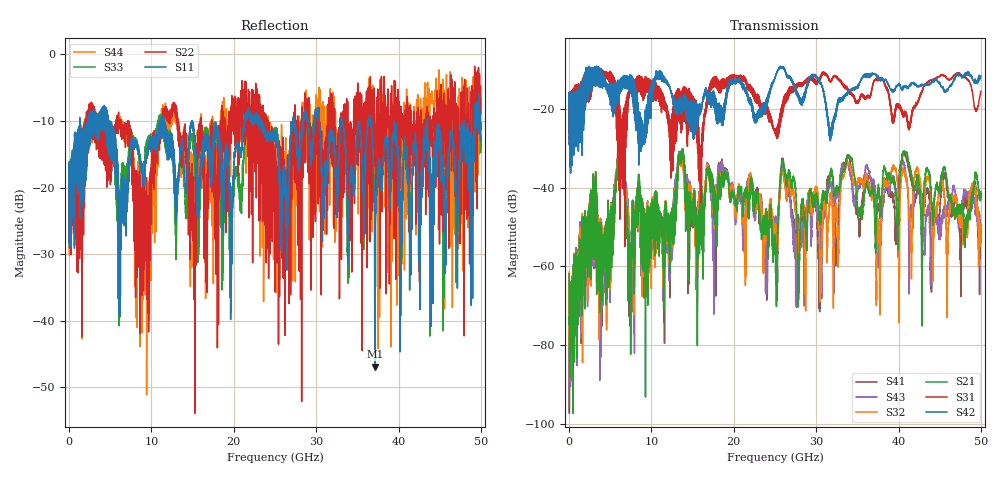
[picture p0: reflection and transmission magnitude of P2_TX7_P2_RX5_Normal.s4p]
!Keysight Technologies,N5225B,MY57041031,A.13.20.10
!Date: Friday, May 31, 2019 11:34:46
!Correction: S11(Full 4 Port(1,2,3,4))
!S12(Full 4 Port(1,2,3,4))
!S13(Full 4 Port(1,2,3,4))
!S14(Full 4 Port(1,2,3,4))
!S21(Full 4 Port(1,2,3,4))
!S22(Full 4 Port(1,2,3,4))
!S23(Full 4 Port(1,2,3,4))
!S24(Full 4 Port(1,2,3,4))
!S31(Full 4 Port(1,2,3,4))
!S32(Full 4 Port(1,2,3,4))
!S33(Full 4 Port(1,2,3,4))
!S34(Full 4 Port(1,2,3,4))
!S41(Full 4 Port(1,2,3,4))
!S42(Full 4 Port(1,2,3,4))
!S43(Full 4 Port(1,2,3,4))
!S44(Full 4 Port(1,2,3,4))
!S4P File: Measurements: <S11,S12,S13,S14>,
!<S21,S22,S23,S24>,
!<S31,S32,S33,S34>,
!<S41,S42,S43,S44>:
# Hz S  dB  R 50.0
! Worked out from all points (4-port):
!   5000 points, 10 MHz to 50 GHz, reference 50 ohm
!   strongest paths, dB at 10 MHz, 12.51 GHz, 25.01 GHz, 37.51 GHz, 50 GHz:
!     S42: -19.4, -16.9, -11.8, -11.8, -11.6
!     S31: -19.5, -22.4, -25.7, -12.7, -15.5
!     S21: -61.9, -46.8, -53.2, -40.4, -40.9
!     S32: -61.4, -52.2, -50.4, -51.3, -49.6
!     S43: -68.1, -53.6, -51.5, -54.6, -52.1
!     S41: -70.5, -48.0, -52.9, -44.6, -53.8
!   lowest |S11| = -46.9 dB at 37.13 GHz (marker M1), VSWR 1.01, Z = 50.5 - j0.039 ohm
!   |S11| at or under -10 dB: 4.911 GHz to 11.03 GHz (6.119 GHz wide, 76.8 % of centre); 14.92 GHz to 21.26 GHz (6.339 GHz wide, 35 % of centre); 36.73 GHz to 43.5 GHz (6.764 GHz wide, 16.9 % of centre)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
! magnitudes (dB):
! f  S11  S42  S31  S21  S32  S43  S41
! 10 MHz  -20.2  -19.4  -19.5  -61.9  -61.4  -68.1  -70.5
! 6.16 GHz  -26.4  -13.1  -48.0  -30.0  -30.1  -29.6  -29.5
! 7.39 GHz  -16.5  -12.6  -14.6  -54.1  -54.7  -55.3  -56.0
! 13.63 GHz  -13.9  -20.0  -26.1  -31.3  -32.7  -32.2  -31.0
! 23.95 GHz  -12.5  -19.4  -20.9  -45.3  -46.0  -59.9  -56.9
! 37.13 GHz  -46.9  -11.1  -12.5  -47.1  -49.6  -40.1  -40.7
! 50 GHz  -11.2  -11.6  -15.5  -40.9  -49.6  -52.1  -53.8
